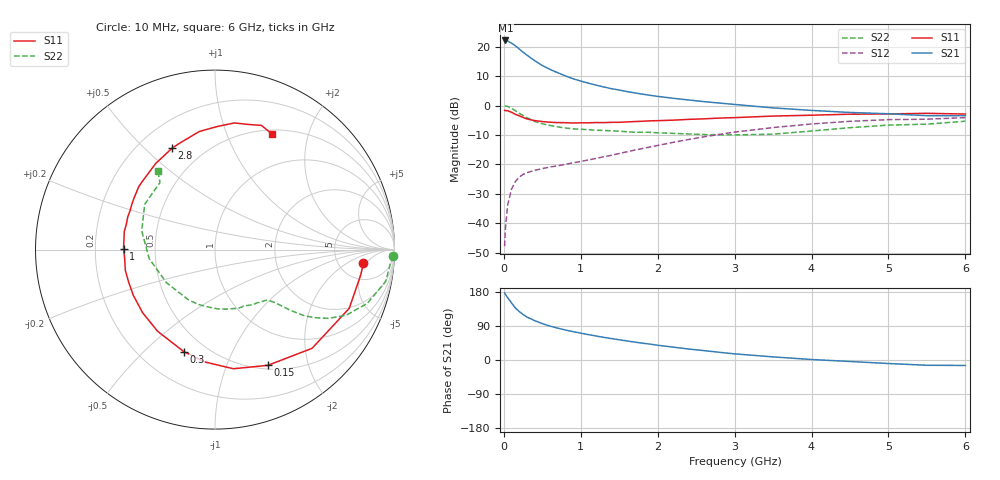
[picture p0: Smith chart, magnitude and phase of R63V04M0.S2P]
! SIEMENS Small Signal Semiconductors
! BFR193
! Si NPN RF Bipolar Junction Transistor in SOT23
! VCE = 3 V  IC = 4 mA
! Common Emitter S-Parameters:  May  1996
# GHz  S  MA  R  50
!  f  S11  S21  S12  S22
! GHz  MAG  ANG  MAG  ANG  MAG  ANG  MAG  ANG
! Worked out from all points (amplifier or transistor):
!   36 points, 10 MHz to 6 GHz, reference 50 ohm
!   highest |S21| = 22.1 dB at 20 MHz (marker M1)
!   |S21| within 3 dB of that: start of sweep to 204.2 MHz
!   unconditionally stable (mu >= 1): 961.8 MHz to 2.01 GHz
!   at 250 MHz: K = 0.37, MSG = 20.7 dB, |S12| = -23.4 dB
!   at 1.4 GHz: K = 1.08, MAG = 9.6 dB, |S12| = -16.9 dB
!   at 6 GHz: K = 0.97, MSG = 0.3 dB, |S12| = -4.1 dB
!   S11 on the Smith chart (normalised r, x): 10 MHz: 8.79, -4.18; 150 MHz: 0.54, -1.41; 300 MHz: 0.38, -0.67; 1 GHz: 0.32, +0.00; 2.8 GHz: 0.34, +0.61; 6 GHz: 0.55, +1.46
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0.01  0.8305 -5.1  12.59 177.1  0.0041 86.5  0.993 -2.1
0.02  0.8242 -9.8  12.76 173.5  0.0081 85.6  0.9814 -4.2
0.05  0.8164 -23.6  12.46 164.3  0.0206 77.1  0.9671 -10.6
0.1  0.7714 -45.5  11.48 150.4  0.0381 67.3  0.9002 -19.4
0.15  0.7087 -65.5  10.37 137.3  0.0512 59.3  0.8169 -26.6
0.2  0.6717 -81.2  9.131 128.0  0.0607 53.6  0.741 -31.1
0.25  0.6284 -95.3  8.039 120.0  0.0678 49.4  0.6755 -34.2
0.3  0.594 -107.1  7.189 113.4  0.0725 46.9  0.6209 -36.5
0.4  0.5561 -125.1  5.807 103.9  0.0795 44.3  0.5405 -38.8
0.5  0.5352 -138.9  4.781 96.0  0.0851 43.7  0.4909 -40.1
0.6  0.5215 -150.8  4.114 89.5  0.0905 44.3  0.4596 -41.0
0.8  0.5127 -167.0  3.195 79.2  0.1006 47.0  0.4162 -43.2
1  0.5097 179.5  2.606 70.8  0.1127 50.7  0.3962 -46.0
1.1  0.51 173.9  2.402 67.0  0.1197 52.4  0.3894 -48.1
1.3  0.5137 164.2  2.068 59.7  0.1352 55.2  0.3773 -52.1
1.6  0.5276 151.4  1.732 50.3  0.1641 58.1  0.3599 -59.9
2.2  0.5653 130.7  1.331 34.0  0.2375 58.2  0.3373 -79.6
2.8  0.6131 113.1  1.104 20.4  0.324 52.6  0.3194 -106.6
3.5  0.6636 97.6  0.914 8.2  0.4233 41.5  0.3274 -145.7
4.5  0.7138 81.3  0.764 -3.9  0.5409 23.9  0.4217 165.6
5.5  0.7388 69.5  0.674 -13.9  0.587 6.1  0.4838 129.3
6  0.7183 63.8  0.676 -14.4  0.6245 1.1  0.5433 125.9
